(* Logix 5000 AddOnInstructionDefinition export AMCI_ANG1E_Resume; software revision 20.05 *)

ADD_ON_INSTRUCTION AMCI_ANG1E_Resume   (* revision 2.0, vendor AMCI *)
// Revision note:
// Version 1.1 added the slot_axis number and the input parameters can now be tags or discrete values.
// 12/4/2023, revision 2.0: Modified AOI so it only writes to output words 0 and 1.
VAR_INPUT
   slot_axis_number : INT; {required}
END_VAR
VAR_IN_OUT
   AMCI_ANG1E_output_data : INT[10]; {required}
END_VAR
VAR
   command_data_block : INT[10];
        [0]   // Command Bits MSW
        [1]   // Command Bits LSW
        [2]   // Upper Target Position
        [3]   // Lower Target Position
        [4]   // Upper Programmed Speed
        [5]   // Lower Programmed Speed
   index : INT;
END_VAR

ROUTINE Logic   (* ladder *)
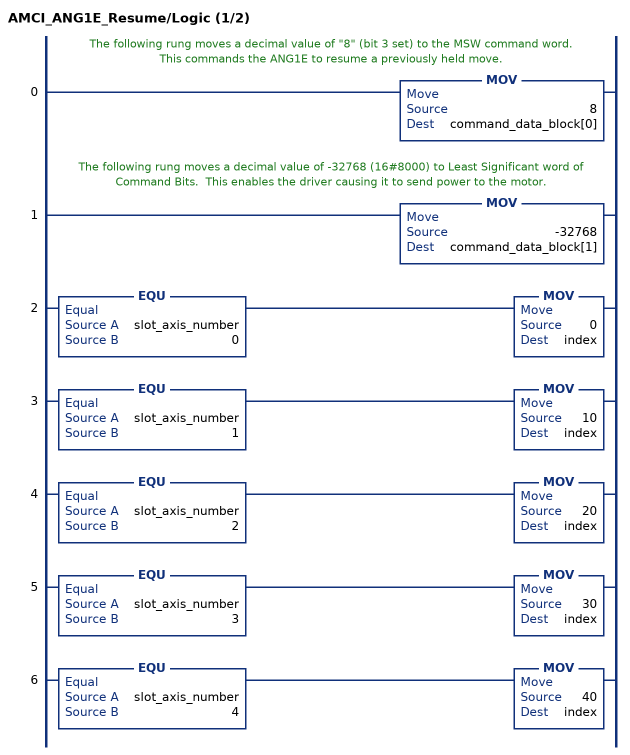
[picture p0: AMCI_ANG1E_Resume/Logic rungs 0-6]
   // The following rung moves a decimal value of "8" (bit 3 set) to the MSW command word.  This commands the ANG1E to resume a previously held move.
   0: MOV(8,command_data_block[0]);
   // The following rung moves a decimal value of -32768 (16#8000) to Least Significant word of Command Bits.  This enables the driver causing it to send power to the motor.
   1: MOV(-32768,command_data_block[1]);
   2: EQU(slot_axis_number,0)MOV(0,index);
   3: EQU(slot_axis_number,1)MOV(10,index);
   4: EQU(slot_axis_number,2)MOV(20,index);
   5: EQU(slot_axis_number,3)MOV(30,index);
   6: EQU(slot_axis_number,4)MOV(40,index);
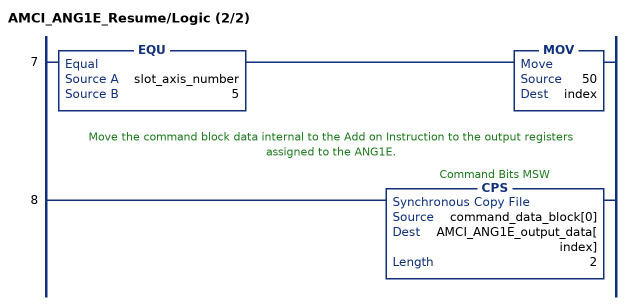
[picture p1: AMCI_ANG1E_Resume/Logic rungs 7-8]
   7: EQU(slot_axis_number,5)MOV(50,index);
   // Move the command block data internal to the Add on Instruction to the output registers assigned to the ANG1E.
   8: CPS(command_data_block[0],AMCI_ANG1E_output_data[index],2);
END_ROUTINE
END_ADD_ON_INSTRUCTION
